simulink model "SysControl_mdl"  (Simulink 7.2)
settings: Solver=ode45  StartTime=0.0  StopTime=10.0  RelTol=1e-3
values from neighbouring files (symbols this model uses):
  A = [ -b1/Ma  -K   b1/Mr         0    [Esercitazione05.m]
  B = [1    [Esercitazione05.m]
  Bd = [-Ma    0    [Esercitazione05.m]
  C = [1/Ma  0   0  0]    [Esercitazione05.m]
  g = 9.81    [Esercitazione05.m]
  Kcontr = -acker(A,B,P)    [Esercitazione05.m]
  X0 = [0 0.05 0 0]'    [Esercitazione05.m]

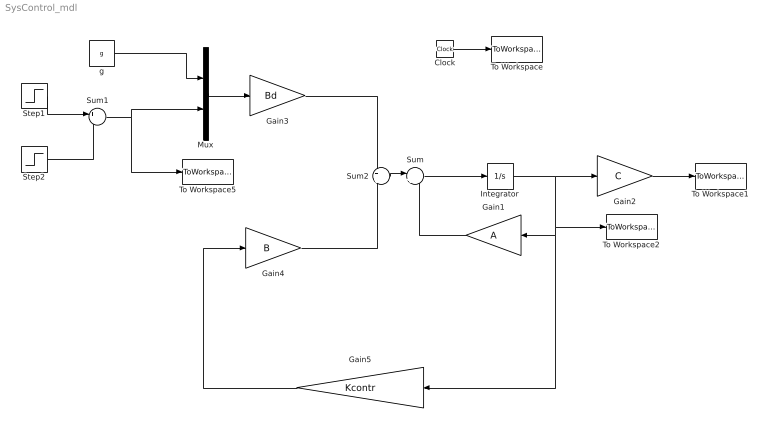
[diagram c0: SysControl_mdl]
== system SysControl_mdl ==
  Clock : Clock
  Gain1 : Gain  Orientation=left  Gain=A  Multiplication=Matrix(K*u)  ParameterDataType=sfix(16)  ParameterScaling=2^0  OutDataType=sfix(16)  OutScaling=2^0
  Gain2 : Gain  Gain=C  Multiplication=Matrix(K*u)  ParameterDataType=sfix(16)  ParameterScaling=2^0  OutDataType=sfix(16)  OutScaling=2^0
  Gain3 : Gain  Gain=Bd  Multiplication=Matrix(K*u)  ParameterDataType=sfix(16)  ParameterScaling=2^0  OutDataType=sfix(16)  OutScaling=2^0
  Gain4 : Gain  Gain=B  Multiplication=Matrix(K*u)  ParameterDataType=sfix(16)  ParameterScaling=2^0  OutDataType=sfix(16)  OutScaling=2^0
  Gain5 : Gain  Orientation=left  Gain=Kcontr  Multiplication=Matrix(K*u)  ParameterDataType=sfix(16)  ParameterScaling=2^0  OutDataType=sfix(16)  OutScaling=2^0
  Integrator : Integrator  InitialCondition=X0
  Mux : Mux  Inputs=2
  Step1 : Step  Time=5  SampleTime=0
  Step2 : Step  Time=5+0.2  SampleTime=0
  Sum : Sum  Inputs=|++  OutDataType=sfix(16)  OutScaling=2^0
  Sum1 : Sum  Inputs=+-  OutDataType=sfix(16)  OutScaling=2^0
  Sum2 : Sum  OutDataType=sfix(16)  OutScaling=2^0
  To Workspace : ToWorkspace  VariableName=time  SampleTime=-1  SaveFormat=Array
  To Workspace1 : ToWorkspace  VariableName=y  SampleTime=-1  SaveFormat=Array
  To Workspace2 : ToWorkspace  VariableName=x  SampleTime=-1  SaveFormat=Array
  To Workspace5 : ToWorkspace  VariableName=dXs  SampleTime=-1  SaveFormat=Array
  g : Constant  Value=g  OutDataType=sfix(16)  OutScaling=2^0
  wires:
  Gain1/1 -> Sum/2
  Sum/1 -> Integrator/1
  Integrator/1 -> Gain2/1, To Workspace2/1, Gain1/1, Gain5/1
  Clock/1 -> To Workspace/1
  Gain2/1 -> To Workspace1/1
  Mux/1 -> Gain3/1
  g/1 -> Mux/1
  Step1/1 -> Sum1/1
  Step2/1 -> Sum1/2
  Sum2/1 -> Sum/1
  Sum1/1 -> Mux/2, To Workspace5/1
  Gain3/1 -> Sum2/1
  Gain4/1 -> Sum2/2
  Gain5/1 -> Gain4/1
